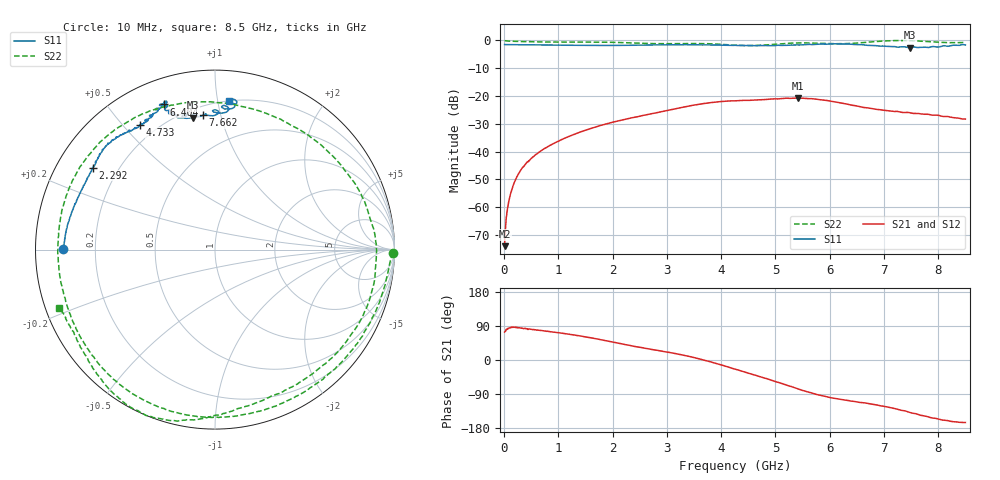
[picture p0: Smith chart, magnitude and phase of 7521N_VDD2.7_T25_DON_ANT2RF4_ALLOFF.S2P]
!Agilent Technologies,E5071C,MY46417908,A.11.23
!Date: Thu Jul 30 15:14:12 2020
!Data & Calibration Information:
!Freq	S11:SOLT2(ON)	S21:SOLT2(ON)	S12:SOLT2(ON)	S22:SOLT2(ON)
!PortZ  Port1:50+j0  Port2:50+j0
!Above PortZ is port z conversion or system Z0 setting when saving the data.
!When reading, reference impedance value at option line is always used.
# Hz S dB R 50
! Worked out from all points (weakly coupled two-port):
!   1601 points, 10 MHz to 8.5 GHz, reference 50 ohm
!   highest |S21| = -20.69 dB at 5.417 GHz (marker M1); lowest = -74.0 dB at 10 MHz (marker M2)
!   lowest |S11| = -2.6 dB at 7.476 GHz (marker M3), VSWR 6.86, Z = 12.3 + j40.8 ohm
!   |S11| at or under -10 dB: nowhere
!   |S22| runs from -1.8 to 0.0 dB; largest |S21 - S12| = 0.0022
!   S11 on the Smith chart (normalised r, x): 10 MHz: 0.08, +0.00; 2.292 GHz: 0.11, +0.30; 4.733 GHz: 0.14, +0.56; 6.404 GHz: 0.12, +0.70; 7.662 GHz: 0.26, +0.88; 8.5 GHz: 0.20, +1.08
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1e7  -1.45 179.9  -74.02 73.9  -73.16 72.7  -0.06 -1.0
7.3675e7  -1.49 178.9  -59.37 83.9  -59.59 83.1  -0.22 -5.4
1.214312e8  -1.49 178.2  -55.05 85.4  -55.14 85.5  -0.26 -8.5
3.28375e8  -1.53 175.2  -46.10 84.3  -46.06 84.2  -0.37 -21.6
8.749188e8  -1.63 167.3  -37.47 74.2  -37.48 74.2  -0.58 -54.5
1.426769e9  -1.77 158.8  -32.78 63.0  -32.80 62.7  -0.59 -85.6
1.851269e9  -1.79 151.6  -30.19 51.6  -30.21 51.4  -0.62 -109.6
2.291688e9  -1.73 146.1  -28.11 39.1  -28.11 39.1  -0.83 -135.1
2.843538e9  -1.57 140.4  -25.85 25.0  -25.86 24.8  -1.14 -166.8
3.565188e9  -1.53 133.2  -23.03 4.3  -23.03 4.3  -1.09 148.9
3.95785e9  -1.68 129.2  -22.04 -11.2  -22.05 -11.3  -1.33 118.9
4.255e9  -1.73 125.8  -21.72 -24.2  -21.72 -24.2  -1.68 93.2
4.732562e9  -1.83 121.1  -21.33 -44.8  -21.30 -45.0  -1.69 50.5
5.098694e9  -1.76 118.4  -20.93 -60.9  -20.89 -60.9  -1.18 18.8
5.417069e9  -1.60 114.4  -20.69 -75.9  -20.66 -75.9  -0.90 -7.6
5.671769e9  -1.48 111.9  -20.95 -87.0  -20.91 -87.2  -0.92 -28.3
6.021981e9  -1.25 108.1  -21.85 -99.7  -21.79 -99.9  -1.13 -54.4
6.404031e9  -1.34 109.3  -23.26 -108.3  -23.20 -108.1  -1.02 -77.8
7.088538e9  -2.15 106.3  -25.32 -124.8  -25.14 -123.3  -0.11 -105.9
7.475894e9  -2.55 99.6  -26.00 -138.4  -25.92 -136.0  -0.06 -120.4
7.661612e9  -2.49 95.1  -26.36 -145.3  -26.33 -143.0  -0.23 -127.7
8.5e9  -1.61 84.6  -28.28 -165.0  -28.35 -165.3  -0.67 -159.4
